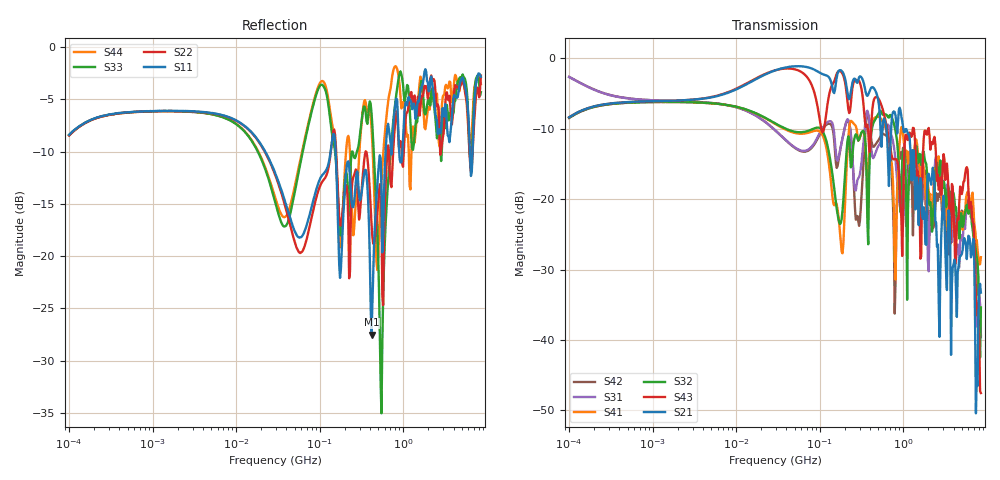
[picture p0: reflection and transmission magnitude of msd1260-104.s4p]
# MHz S MA R 50
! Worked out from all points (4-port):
!   498 points, 100 kHz to 8.5 GHz, reference 50 ohm
!   strongest paths, dB at 100 kHz, 1.698 MHz, 29.49 MHz, 500.7 MHz, 8.5 GHz:
!     S21: -8.4, -6.0, -1.7, -5.9, -33.3
!     S43: -8.4, -6.0, -1.7, -5.7, -47.5
!     S32: -8.5, -6.2, -9.3, -7.9, -35.4
!     S41: -8.5, -6.2, -9.3, -8.3, -28.2
!     S31: -2.7, -6.1, -10.2, -12.5, -39.6
!     S42: -2.6, -6.1, -10.3, -11.7, -39.3
!   lowest |S11| = -27.5 dB at 417.1 MHz (marker M1), VSWR 1.09, Z = 53.7 - j2.31 ohm
!   |S11| at or under -10 dB: 22.28 MHz to 135.1 MHz (112.8 MHz wide, 143 % of centre); 154.9 MHz to 614.7 MHz (459.8 MHz wide, 119 % of centre); 6.277 GHz to 6.758 GHz (481.1 MHz wide, 7.38 % of centre)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
0.1  0.3803 38.5  0.381 39.1  0.7354 -19.0  0.3773 -141.6
     0.381 39.1  0.3775 38.4  0.3776 -141.5  0.7382 -19.1
     0.7354 -19.0  0.3776 -141.5  0.3808 38.6  0.3807 38.9
     0.3773 -141.6  0.7382 -19.1  0.3807 38.9  0.3785 38.5
417.0585  0.04203 -30.7  0.6214 -80.6  0.2197 -25.2  0.3421 4.2
          0.6214 -80.6  0.1429 -63.6  0.304 24.2  0.2567 -18.5
          0.2197 -25.2  0.304 24.2  0.4839 -100.3  0.3623 -42.9
          0.3421 4.2  0.2567 -18.5  0.3623 -42.9  0.4126 -110.2
548.5512  0.214 -58.2  0.2354 -106.1  0.2812 -27.6  0.3656 -60.1
          0.2354 -106.1  0.1621 -79.6  0.4139 -40.2  0.2879 -44.7
          0.2812 -27.6  0.4139 -40.2  0.01768 88.0  0.4633 -103.1
          0.3656 -60.1  0.2879 -44.7  0.4633 -103.1  0.229 35.5
906.6107  0.2909 -96.5  0.4461 -130.1  0.08982 -136.8  0.2539 -46.3
          0.4461 -130.1  0.3346 -83.2  0.1198 -143.5  0.2109 -59.9
          0.08982 -136.8  0.1198 -143.5  0.7533 -76.3  0.1279 -154.3
          0.2539 -46.3  0.2109 -59.9  0.1279 -154.3  0.6532 -118.9
3111.8  0.4664 65.6  0.07633 110.9  0.09196 45.2  0.07813 35.6
        0.07633 110.9  0.4407 82.9  0.1285 37.0  0.07483 30.0
        0.09196 45.2  0.1285 37.0  0.4678 71.3  0.1921 3.4
        0.07813 35.6  0.07483 30.0  0.1921 3.4  0.597 83.3
5765.102  0.5791 -128.4  0.03756 54.8  0.08754 174.3  0.1085 -175.7
          0.03756 54.8  0.5464 -133.1  0.09132 166.9  0.09074 173.6
          0.08754 174.3  0.09132 166.9  0.6207 -127.7  0.1687 42.3
          0.1085 -175.7  0.09074 173.6  0.1687 42.3  0.5315 -126.9
8500  0.7223 -54.2  0.02173 -68.8  0.01044 128.9  0.03872 -105.7
      0.02173 -68.8  0.7325 -41.2  0.01702 -48.7  0.01081 -117.5
      0.01044 128.9  0.01702 -48.7  0.609 -40.0  0.004203 -180.0
      0.03872 -105.7  0.01081 -117.5  0.004203 -180.0  0.6671 -55.2
